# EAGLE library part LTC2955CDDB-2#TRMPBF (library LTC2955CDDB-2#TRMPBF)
Pushbutton On/Off Controller with Automatic Turn-On Source: Datasheet
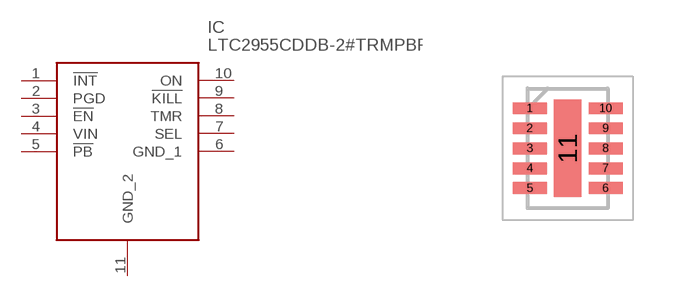
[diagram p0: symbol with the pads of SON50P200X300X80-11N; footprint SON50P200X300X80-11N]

Designator prefix IC

## LTC2955CDDB-2#TRMPBF (Arrow_Part_Number: LTC2955CDDB-2#TRMPBF; Arrow_Price-Stock: https://www.arrow.com/en/products/ltc2955cddb-2trmpbf/linear-technology; Description: Pushbutton On/Off Controller with Automatic Turn-On; Height: 0.8mm; Manufacturer_Name: Analog Devices; Manufacturer_Part_Number: LTC2955CDDB-2#TRMPBF; Mouser_Part_Number: 584-C2955CDDB-2TMPF; Mouser_Price-Stock: https://www.mouser.co.uk/ProductDetail/Analog-Devices/LTC2955CDDB-2TRMPBF?qs=hVkxg5c3xu85EnUZHVDmnw%3D%3D)  [SON50P200X300X80-11N]
1  !INT
2  PGD
3  !EN
4  VIN
5  !PB
6  GND_1
7  SEL
8  TMR
9  !KILL
10  ON
11  GND_2

## Footprint SON50P200X300X80-11N (pad centres in mm)
10-Lead Plastic DFN (3mm &times; 2mm)
smd 0.85 x 0.3: 1 -0.95,1; 2 -0.95,0.5; 3 -0.95,0; 4 -0.95,-0.5; 5 -0.95,-1; 6 0.95,-1; 7 0.95,-0.5; 8 0.95,0; 9 0.95,0.5; 10 0.95,1
smd 0.69 x 2.44: 11 0,0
